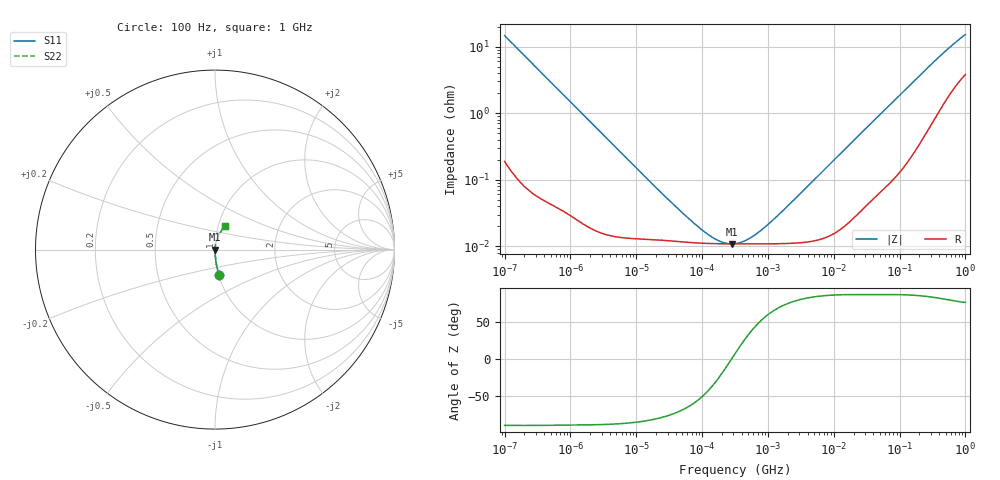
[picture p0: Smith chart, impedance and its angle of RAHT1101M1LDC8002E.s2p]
! RAHT1101M1LDC8002E  S-PARAMETER MODEL  (AEC-Q200 qualified)
! Model Generated by ELNA Corporation (http://www.ty-top.com)
! Version 1.0
! ELNA Control No. 240229
! Copyright (c) 2024 ELNA CO.,LTD. All Rights Reserved.
! Products Name : CONDUCTIVE POLYMER HYBRID ALUMINUM ELECTROLYTIC CAPACITORS
! Characteristics :
!  Capacitance  :  100uF  ,  Rated voltage  :  10V
!  Operating Temp. Range  :  -55 to +105 degC  ,  Endurance  :  10000hr at 105 degC
!  Dimension D  :  6.3mm  ,  Dimension L  :  5.8mm
! Frequency Range : 100Hz - 1GHz
! External Node Assignments :
!  1  o---| |---o  2
# MHz S RI R 50
!Freq[MHz].  S11 Real  S11 Imag  S21 Real  S21 Imag  S12 Real  S12 Imag  S22 Real  S22 Imag
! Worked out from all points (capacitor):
!   401 points, 100 Hz to 1 GHz, reference 50 ohm
!   read as one part in series: C = 109 uF near 108 Hz
!   lowest |Z| = 10.9 mohm at 280.2 kHz (marker M1)
!   series resonance near 281.8 kHz, so ESL is about 2.9 nH
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0.0001  0.0227 -0.1426  0.9773 0.1426  0.9773 0.1426  0.0227 -0.1426
0.000113  0.018 -0.127  0.982 0.127  0.982 0.127  0.018 -0.127
0.000183  0.00719 -0.0793  0.9928 0.0793  0.9928 0.0793  0.00719 -0.0793
0.000309  0.0028 -0.0472  0.9972 0.0472  0.9972 0.0472  0.0028 -0.0472
0.001488  0.000322 -0.00996  0.9997 0.00996  0.9997 0.00996  0.000322 -0.00996
0.022131  0.000125 -0.000677  0.9999 0.000677  0.9999 0.000677  0.000125 -0.000677
0.060604  0.000115 -0.000243  0.9999 0.000243  0.9999 0.000243  0.000115 -0.000243
0.115478  0.000111 -0.000112  0.9999 0.000112  0.9999 0.000112  0.000111 -0.000112
0.187284  0.000109 -4.67e-05  0.9999 4.67e-05  0.9999 4.67e-05  0.000109 -4.67e-05
0.229087  0.000109 -2.32e-05  0.9999 2.32e-05  0.9999 2.32e-05  0.000109 -2.32e-05
0.280221  0.000109 -6.03e-07  0.9999 6.03e-07  0.9999 6.03e-07  0.000109 -6.03e-07
0.316228  0.000109 1.29e-05  0.9999 -1.29e-05  0.9999 -1.29e-05  0.000109 1.29e-05
0.386812  0.000109 3.59e-05  0.9999 -3.59e-05  0.9999 -3.59e-05  0.000109 3.59e-05
0.492606  0.000109 6.56e-05  0.9999 -6.56e-05  0.9999 -6.56e-05  0.000109 6.56e-05
0.798914  0.000109 0.000138  0.9999 -0.000138  0.9999 -0.000138  0.000109 0.000138
1.522299  0.00011 0.000291  0.9999 -0.000291  0.9999 -0.000291  0.00011 0.000291
4.704354  0.00012 0.000926  0.9999 -0.000926  0.9999 -0.000926  0.00012 0.000926
69.9842  0.00104 0.013  0.999 -0.013  0.999 -0.013  0.00104 0.013
176.8072  0.00381 0.0319  0.9962 -0.0319  0.9962 -0.0319  0.00381 0.0319
395.8221  0.0149 0.067  0.9851 -0.067  0.9851 -0.067  0.0149 0.067
695.825  0.0354 0.1047  0.9646 -0.1047  0.9646 -0.1047  0.0354 0.1047
1000  0.0555 0.1339  0.9445 -0.1339  0.9445 -0.1339  0.0555 0.1339
